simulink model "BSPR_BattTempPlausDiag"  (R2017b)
settings: Solver=FixedStepDiscrete  StartTime=0.0  StopTime=10.0  FixedStep=0.02  RelTol=1e-3  EnableMultiTasking=on
undefined symbols (not defined in the file): bin2dec, BSPR_cntBattTCnstErrDet_C, BSPR_cntBattTCnstErrHeal_C, BSPR_cntBattTHopErrDet_C, BSPR_cntBattTHopErrHeal_C, BSPR_cntBattTPlausDiag_CW, BSPR_cntCellTPlausDiag_CW, BSPR_cofBattTLowPassK_C, BSPR_tBattTCnstFaultThres_C, BSPR_tBattTempCnstHi_C, BSPR_tBattTempCnstLo_C, BSPR_tBattTempCnstThres_C, BSPR_tBattTempEnvtDiff_C, BSPR_tBattTHopFaultThres_C, BSPR_tBusbarTCnstFaultThres_C, BSPR_tBusbarTCnstHealThres_C, BSPR_tCellTCnstFaultThres_C, BSPR_tCellTCnstHealThres_C, BSPR_tiBattTCnstErrDet_C, BSPR_tiBattTCnstErrHeal_C
libraries: simulink x12
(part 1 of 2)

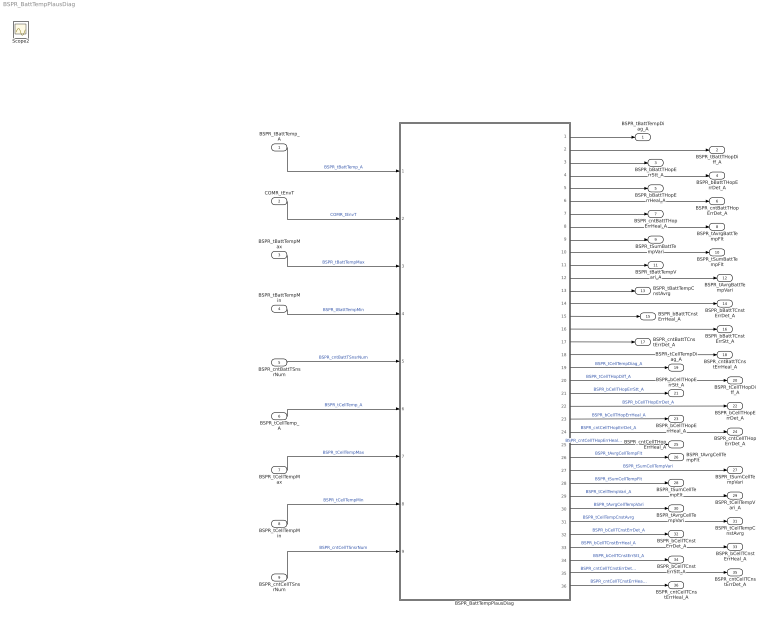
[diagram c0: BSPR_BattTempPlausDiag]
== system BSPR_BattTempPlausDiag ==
  BSPR_tBattTemp_A : Inport
  COMR_tEnvT : Inport  Port=2
  BSPR_tBattTempMax : Inport  Port=3
  BSPR_tBattTempMin : Inport  Port=4
  BSPR_cntBattTSnsrNum : Inport  Port=5
  BSPR_tCellTemp_A : Inport  Port=6
  BSPR_tCellTempMax : Inport  Port=7
  BSPR_tCellTempMin : Inport  Port=8
  BSPR_cntCellTSnsrNum : Inport  Port=9
  BSPR_BattTempPlausDiag : Subsystem
  BSPR_tBattTempDiag_A : Outport
  BSPR_tBattTHopDiff_A : Outport  Port=2
  BSPR_bBattTHopErrStt_A : Outport  Port=3
  BSPR_bBattTHopErrDet_A : Outport  Port=4
  BSPR_bBattTHopErrHeal_A : Outport  Port=5
  BSPR_cntBattTHopErrDet_A : Outport  Port=6
  BSPR_cntBattTHopErrHeal_A : Outport  Port=7
  BSPR_tAvrgBattTempFlt : Outport  Port=8
  BSPR_tSumBattTempVari : Outport  Port=9
  BSPR_tSumBattTempFlt : Outport  Port=10
  BSPR_tBattTempVari_A : Outport  Port=11
  BSPR_tAvrgBattTempVari : Outport  Port=12
  BSPR_tBattTempCnstAvrg : Outport  Port=13
  BSPR_bBattTCnstErrDet_A : Outport  Port=14
  BSPR_bBattTCnstErrHeal_A : Outport  Port=15
  BSPR_bBattTCnstErrStt_A : Outport  Port=16
  BSPR_cntBattTCnstErrDet_A : Outport  Port=17
  BSPR_cntBattTCnstErrHeal_A : Outport  Port=18
  BSPR_tCellTempDiag_A : Outport  Port=19  InitialOutput=[0]
  BSPR_tCellTHopDiff_A : Outport  Port=20  InitialOutput=[0]
  BSPR_bCellTHopErrStt_A : Outport  Port=21  InitialOutput=[0]
  BSPR_bCellTHopErrDet_A : Outport  Port=22
  BSPR_bCellTHopErrHeal_A : Outport  Port=23
  BSPR_cntCellTHopErrDet_A : Outport  Port=24  InitialOutput=[0]
  BSPR_cntCellTHopErrHeal_A : Outport  Port=25  InitialOutput=[0]
  BSPR_tAvrgCellTempFlt : Outport  Port=26  InitialOutput=[0]
  BSPR_tSumCellTempVari : Outport  Port=27  InitialOutput=[0]
  BSPR_tSumCellTempFlt : Outport  Port=28  InitialOutput=[0]
  BSPR_tCellTempVari_A : Outport  Port=29  InitialOutput=[0]
  BSPR_tAvrgCellTempVari : Outport  Port=30  InitialOutput=[0]
  BSPR_tCellTempCnstAvrg : Outport  Port=31  InitialOutput=[0]
  BSPR_bCellTCnstErrDet_A : Outport  Port=32  InitialOutput=[0]
  BSPR_bCellTCnstErrHeal_A : Outport  Port=33  InitialOutput=[0]
  BSPR_bCellTCnstErrStt_A : Outport  Port=34  InitialOutput=[0]
  BSPR_cntCellTCnstErrDet_A : Outport  Port=35  InitialOutput=[0]
  BSPR_cntCellTCnstErrHeal_A : Outport  Port=36  InitialOutput=[0]
  Scope2 : Scope
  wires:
  BSPR_tBattTemp_A/1 -> BSPR_BattTempPlausDiag/1(BSPR_tBattTemp_A)  "BSPR_tBattTemp_A"
  COMR_tEnvT/1 -> BSPR_BattTempPlausDiag/2(COMR_tEnvT)  "COMR_tEnvT"
  BSPR_tBattTempMax/1 -> BSPR_BattTempPlausDiag/3(BSPR_tBattTempMax)  "BSPR_tBattTempMax"
  BSPR_tBattTempMin/1 -> BSPR_BattTempPlausDiag/4(BSPR_tBattTempMin)  "BSPR_tBattTempMin"
  BSPR_BattTempPlausDiag/1(BSPR_tBattTempDiag_A) -> BSPR_tBattTempDiag_A/1
  BSPR_BattTempPlausDiag/2(BSPR_tBattTHopDiff_A) -> BSPR_tBattTHopDiff_A/1
  BSPR_BattTempPlausDiag/3(BSPR_bBattTHopErrStt_A) -> BSPR_bBattTHopErrStt_A/1
  BSPR_BattTempPlausDiag/4(BSPR_bBattTHopErrDet_A) -> BSPR_bBattTHopErrDet_A/1
  BSPR_BattTempPlausDiag/5(BSPR_bBattTHopErrHeal_A) -> BSPR_bBattTHopErrHeal_A/1
  BSPR_BattTempPlausDiag/6(BSPR_cntBattTHopErrDet_A) -> BSPR_cntBattTHopErrDet_A/1
  BSPR_BattTempPlausDiag/7(BSPR_cntBattTHopErrHeal_A) -> BSPR_cntBattTHopErrHeal_A/1
  BSPR_BattTempPlausDiag/8(BSPR_tAvrgBattTempFlt) -> BSPR_tAvrgBattTempFlt/1
  BSPR_BattTempPlausDiag/9(BSPR_tSumBattTempVari) -> BSPR_tSumBattTempVari/1
  BSPR_BattTempPlausDiag/10(BSPR_tSumBattTempFlt) -> BSPR_tSumBattTempFlt/1
  BSPR_BattTempPlausDiag/11(BSPR_tBattTempVari_A) -> BSPR_tBattTempVari_A/1
  BSPR_BattTempPlausDiag/12(BSPR_tAvrgBattTempVari) -> BSPR_tAvrgBattTempVari/1
  BSPR_BattTempPlausDiag/13(BSPR_tBattTempCnstAvrg) -> BSPR_tBattTempCnstAvrg/1
  BSPR_BattTempPlausDiag/14(BSPR_bBattTCnstErrDet_A) -> BSPR_bBattTCnstErrDet_A/1
  BSPR_BattTempPlausDiag/15(BSPR_bBattTCnstErrHeal_A) -> BSPR_bBattTCnstErrHeal_A/1
  BSPR_BattTempPlausDiag/16(BSPR_bBattTCnstErrStt_A) -> BSPR_bBattTCnstErrStt_A/1
  BSPR_BattTempPlausDiag/17(BSPR_cntBattTCnstErrDet_A) -> BSPR_cntBattTCnstErrDet_A/1
  BSPR_BattTempPlausDiag/18(BSPR_cntBattTCnstErrHeal_A) -> BSPR_cntBattTCnstErrHeal_A/1
  BSPR_cntBattTSnsrNum/1 -> BSPR_BattTempPlausDiag/5(BSPR_cntBattTSnsrNum)  "BSPR_cntBattTSnsrNum"
  BSPR_tCellTemp_A/1 -> BSPR_BattTempPlausDiag/6(BSPR_tCellTemp_A)  "BSPR_tCellTemp_A"
  BSPR_tCellTempMax/1 -> BSPR_BattTempPlausDiag/7(BSPR_tCellTempMax)  "BSPR_tCellTempMax"
  BSPR_tCellTempMin/1 -> BSPR_BattTempPlausDiag/8(BSPR_tCellTempMin)  "BSPR_tCellTempMin"
  BSPR_cntCellTSnsrNum/1 -> BSPR_BattTempPlausDiag/9(BSPR_cntCellTSnsrNum)  "BSPR_cntCellTSnsrNum"
  BSPR_BattTempPlausDiag/26(BSPR_tAvrgCellTempFlt) -> BSPR_tAvrgCellTempFlt/1  "BSPR_tAvrgCellTempFlt"
  BSPR_BattTempPlausDiag/30(BSPR_tAvrgCellTempVari) -> BSPR_tAvrgCellTempVari/1  "BSPR_tAvrgCellTempVari"
  BSPR_BattTempPlausDiag/23(BSPR_bCellTHopErrHeal_A) -> BSPR_bCellTHopErrHeal_A/1  "BSPR_bCellTHopErrHeal_A"
  BSPR_BattTempPlausDiag/32(BSPR_bCellTCnstErrDet_A) -> BSPR_bCellTCnstErrDet_A/1  "BSPR_bCellTCnstErrDet_A"
  BSPR_BattTempPlausDiag/36(BSPR_cntCellTCnstErrHeal_A) -> BSPR_cntCellTCnstErrHeal_A/1  "BSPR_cntCellTCnstErrHeal_A"
  BSPR_BattTempPlausDiag/33(BSPR_bCellTCnstErrHeal_A) -> BSPR_bCellTCnstErrHeal_A/1  "BSPR_bCellTCnstErrHeal_A"
  BSPR_BattTempPlausDiag/22(BSPR_bCellTHopErrDet_A) -> BSPR_bCellTHopErrDet_A/1  "BSPR_bCellTHopErrDet_A"
  BSPR_BattTempPlausDiag/29(BSPR_tCellTempVari_A) -> BSPR_tCellTempVari_A/1  "BSPR_tCellTempVari_A"
  BSPR_BattTempPlausDiag/34(BSPR_bCellTCnstErrStt_A) -> BSPR_bCellTCnstErrStt_A/1  "BSPR_bCellTCnstErrStt_A"
  BSPR_BattTempPlausDiag/31(BSPR_tCellTempCnstAvrg) -> BSPR_tCellTempCnstAvrg/1  "BSPR_tCellTempCnstAvrg"
  BSPR_BattTempPlausDiag/24(BSPR_cntCellTHopErrDet_A) -> BSPR_cntCellTHopErrDet_A/1  "BSPR_cntCellTHopErrDet_A"
  BSPR_BattTempPlausDiag/27(BSPR_tSumCellTempVari) -> BSPR_tSumCellTempVari/1  "BSPR_tSumCellTempVari"
  BSPR_BattTempPlausDiag/28(BSPR_tSumCellTempFlt) -> BSPR_tSumCellTempFlt/1  "BSPR_tSumCellTempFlt"
  BSPR_BattTempPlausDiag/35(BSPR_cntCellTCnstErrDet_A) -> BSPR_cntCellTCnstErrDet_A/1  "BSPR_cntCellTCnstErrDet_A"
  BSPR_BattTempPlausDiag/19(BSPR_tCellTempDiag_A) -> BSPR_tCellTempDiag_A/1  "BSPR_tCellTempDiag_A"
  BSPR_BattTempPlausDiag/25(BSPR_cntCellTHopErrHeal_A) -> BSPR_cntCellTHopErrHeal_A/1  "BSPR_cntCellTHopErrHeal_A"
  BSPR_BattTempPlausDiag/20(BSPR_tCellTHopDiff_A) -> BSPR_tCellTHopDiff_A/1  "BSPR_tCellTHopDiff_A"
  BSPR_BattTempPlausDiag/21(BSPR_bCellTHopErrStt_A) -> BSPR_bCellTHopErrStt_A/1  "BSPR_bCellTHopErrStt_A"

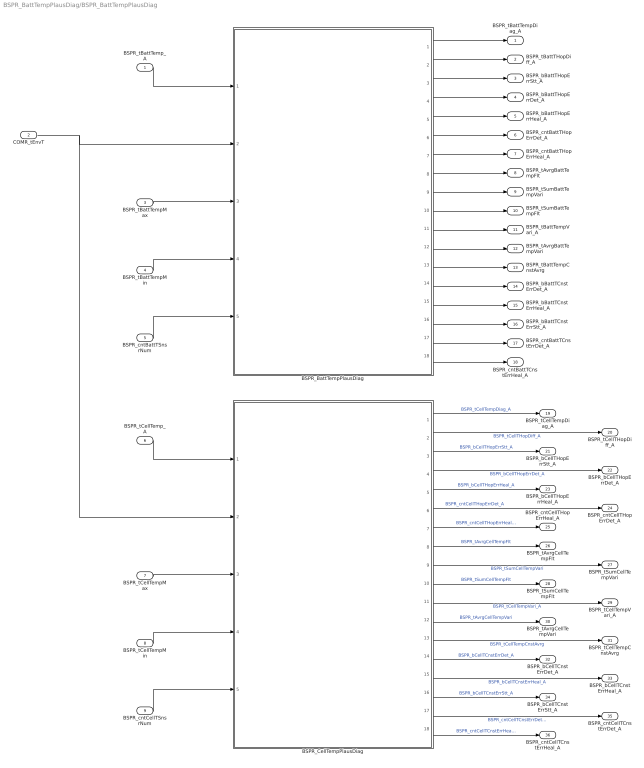
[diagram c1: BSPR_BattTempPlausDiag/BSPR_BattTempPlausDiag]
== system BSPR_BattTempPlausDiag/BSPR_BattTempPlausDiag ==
  BSPR_tBattTemp_A : Inport
  COMR_tEnvT : Inport  Port=2
  BSPR_tBattTempMax : Inport  Port=3
  BSPR_tBattTempMin : Inport  Port=4
  BSPR_cntBattTSnsrNum : Inport  Port=5
  BSPR_tCellTemp_A : Inport  Port=6
  BSPR_tCellTempMax : Inport  Port=7
  BSPR_tCellTempMin : Inport  Port=8
  BSPR_cntCellTSnsrNum : Inport  Port=9
  BSPR_BattTempPlausDiag : Subsystem
  BSPR_CellTempPlausDiag : Subsystem
  BSPR_tBattTempDiag_A : Outport
  BSPR_tBattTHopDiff_A : Outport  Port=2
  BSPR_bBattTHopErrStt_A : Outport  Port=3
  BSPR_bBattTHopErrDet_A : Outport  Port=4
  BSPR_bBattTHopErrHeal_A : Outport  Port=5
  BSPR_cntBattTHopErrDet_A : Outport  Port=6
  BSPR_cntBattTHopErrHeal_A : Outport  Port=7
  BSPR_tAvrgBattTempFlt : Outport  Port=8
  BSPR_tSumBattTempVari : Outport  Port=9
  BSPR_tSumBattTempFlt : Outport  Port=10
  BSPR_tBattTempVari_A : Outport  Port=11
  BSPR_tAvrgBattTempVari : Outport  Port=12
  BSPR_tBattTempCnstAvrg : Outport  Port=13
  BSPR_bBattTCnstErrDet_A : Outport  Port=14
  BSPR_bBattTCnstErrHeal_A : Outport  Port=15
  BSPR_bBattTCnstErrStt_A : Outport  Port=16
  BSPR_cntBattTCnstErrDet_A : Outport  Port=17
  BSPR_cntBattTCnstErrHeal_A : Outport  Port=18
  BSPR_tCellTempDiag_A : Outport  Port=19  InitialOutput=[0]
  BSPR_tCellTHopDiff_A : Outport  Port=20  InitialOutput=[0]
  BSPR_bCellTHopErrStt_A : Outport  Port=21  InitialOutput=[0]
  BSPR_bCellTHopErrDet_A : Outport  Port=22
  BSPR_bCellTHopErrHeal_A : Outport  Port=23
  BSPR_cntCellTHopErrDet_A : Outport  Port=24  InitialOutput=[0]
  BSPR_cntCellTHopErrHeal_A : Outport  Port=25  InitialOutput=[0]
  BSPR_tAvrgCellTempFlt : Outport  Port=26  InitialOutput=[0]
  BSPR_tSumCellTempVari : Outport  Port=27  InitialOutput=[0]
  BSPR_tSumCellTempFlt : Outport  Port=28  InitialOutput=[0]
  BSPR_tCellTempVari_A : Outport  Port=29  InitialOutput=[0]
  BSPR_tAvrgCellTempVari : Outport  Port=30  InitialOutput=[0]
  BSPR_tCellTempCnstAvrg : Outport  Port=31  InitialOutput=[0]
  BSPR_bCellTCnstErrDet_A : Outport  Port=32  InitialOutput=[0]
  BSPR_bCellTCnstErrHeal_A : Outport  Port=33  InitialOutput=[0]
  BSPR_bCellTCnstErrStt_A : Outport  Port=34  InitialOutput=[0]
  BSPR_cntCellTCnstErrDet_A : Outport  Port=35  InitialOutput=[0]
  BSPR_cntCellTCnstErrHeal_A : Outport  Port=36  InitialOutput=[0]
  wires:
  BSPR_tBattTemp_A/1 -> BSPR_BattTempPlausDiag/1(BSPR_tBattTemp_A)
  COMR_tEnvT/1 -> BSPR_CellTempPlausDiag/2(COMR_tEnvT), BSPR_BattTempPlausDiag/2(COMR_tEnvT)
  BSPR_tBattTempMax/1 -> BSPR_BattTempPlausDiag/3(BSPR_tBattTempMax)
  BSPR_tBattTempMin/1 -> BSPR_BattTempPlausDiag/4(BSPR_tBattTempMin)
  BSPR_cntBattTSnsrNum/1 -> BSPR_BattTempPlausDiag/5(BSPR_cntBattTSnsrNum)
  BSPR_BattTempPlausDiag/1(BSPR_tBattTempDiag_A) -> BSPR_tBattTempDiag_A/1
  BSPR_BattTempPlausDiag/2(BSPR_tBattTHopDiff_A) -> BSPR_tBattTHopDiff_A/1
  BSPR_BattTempPlausDiag/3(BSPR_bBattTHopErrStt_A) -> BSPR_bBattTHopErrStt_A/1
  BSPR_BattTempPlausDiag/4(BSPR_bBattTHopErrDet_A) -> BSPR_bBattTHopErrDet_A/1
  BSPR_BattTempPlausDiag/5(BSPR_bBattTHopErrHeal_A) -> BSPR_bBattTHopErrHeal_A/1
  BSPR_BattTempPlausDiag/6(BSPR_cntBattTHopErrDet_A) -> BSPR_cntBattTHopErrDet_A/1
  BSPR_BattTempPlausDiag/7(BSPR_cntBattTHopErrHeal_A) -> BSPR_cntBattTHopErrHeal_A/1
  BSPR_BattTempPlausDiag/8(BSPR_tAvrgBattTempFlt) -> BSPR_tAvrgBattTempFlt/1
  BSPR_BattTempPlausDiag/9(BSPR_tSumBattTempVari) -> BSPR_tSumBattTempVari/1
  BSPR_BattTempPlausDiag/10(BSPR_tSumBattTempFlt) -> BSPR_tSumBattTempFlt/1
  BSPR_BattTempPlausDiag/11(BSPR_tBattTempVari_A) -> BSPR_tBattTempVari_A/1
  BSPR_BattTempPlausDiag/12(BSPR_tAvrgBattTempVari) -> BSPR_tAvrgBattTempVari/1
  BSPR_BattTempPlausDiag/13(BSPR_tBattTempCnstAvrg) -> BSPR_tBattTempCnstAvrg/1
  BSPR_BattTempPlausDiag/14(BSPR_bBattTCnstErrDet_A) -> BSPR_bBattTCnstErrDet_A/1
  BSPR_BattTempPlausDiag/15(BSPR_bBattTCnstErrHeal_A) -> BSPR_bBattTCnstErrHeal_A/1
  BSPR_BattTempPlausDiag/16(BSPR_bBattTCnstErrStt_A) -> BSPR_bBattTCnstErrStt_A/1
  BSPR_BattTempPlausDiag/17(BSPR_cntBattTCnstErrDet_A) -> BSPR_cntBattTCnstErrDet_A/1
  BSPR_BattTempPlausDiag/18(BSPR_cntBattTCnstErrHeal_A) -> BSPR_cntBattTCnstErrHeal_A/1
  BSPR_cntCellTSnsrNum/1 -> BSPR_CellTempPlausDiag/5(BSPR_cntCellTSnsrNum)
  BSPR_tCellTempMin/1 -> BSPR_CellTempPlausDiag/4(BSPR_tCellTempMin)
  BSPR_tCellTempMax/1 -> BSPR_CellTempPlausDiag/3(BSPR_tCellTempMax)
  BSPR_tCellTemp_A/1 -> BSPR_CellTempPlausDiag/1(BSPR_tCellTemp_A)
  BSPR_CellTempPlausDiag/8(BSPR_tAvrgCellTempFlt) -> BSPR_tAvrgCellTempFlt/1  "BSPR_tAvrgCellTempFlt"
  BSPR_CellTempPlausDiag/15(BSPR_bCellTCnstErrHeal_A) -> BSPR_bCellTCnstErrHeal_A/1  "BSPR_bCellTCnstErrHeal_A"
  BSPR_CellTempPlausDiag/12(BSPR_tAvrgCellTempVari) -> BSPR_tAvrgCellTempVari/1  "BSPR_tAvrgCellTempVari"
  BSPR_CellTempPlausDiag/13(BSPR_tCellTempCnstAvrg) -> BSPR_tCellTempCnstAvrg/1  "BSPR_tCellTempCnstAvrg"
  BSPR_CellTempPlausDiag/11(BSPR_tCellTempVari_A) -> BSPR_tCellTempVari_A/1  "BSPR_tCellTempVari_A"
  BSPR_CellTempPlausDiag/16(BSPR_bCellTCnstErrStt_A) -> BSPR_bCellTCnstErrStt_A/1  "BSPR_bCellTCnstErrStt_A"
  BSPR_CellTempPlausDiag/4(BSPR_bCellTHopErrDet_A) -> BSPR_bCellTHopErrDet_A/1  "BSPR_bCellTHopErrDet_A"
  BSPR_CellTempPlausDiag/14(BSPR_bCellTCnstErrDet_A) -> BSPR_bCellTCnstErrDet_A/1  "BSPR_bCellTCnstErrDet_A"
  BSPR_CellTempPlausDiag/5(BSPR_bCellTHopErrHeal_A) -> BSPR_bCellTHopErrHeal_A/1  "BSPR_bCellTHopErrHeal_A"
  BSPR_CellTempPlausDiag/18(BSPR_cntCellTCnstErrHeal_A) -> BSPR_cntCellTCnstErrHeal_A/1  "BSPR_cntCellTCnstErrHeal_A"
  BSPR_CellTempPlausDiag/3(BSPR_bCellTHopErrStt_A) -> BSPR_bCellTHopErrStt_A/1  "BSPR_bCellTHopErrStt_A"
  BSPR_CellTempPlausDiag/7(BSPR_cntCellTHopErrHeal_A) -> BSPR_cntCellTHopErrHeal_A/1  "BSPR_cntCellTHopErrHeal_A"
  BSPR_CellTempPlausDiag/1(BSPR_tCellTempDiag_A) -> BSPR_tCellTempDiag_A/1  "BSPR_tCellTempDiag_A"
  BSPR_CellTempPlausDiag/6(BSPR_cntCellTHopErrDet_A) -> BSPR_cntCellTHopErrDet_A/1  "BSPR_cntCellTHopErrDet_A"
  BSPR_CellTempPlausDiag/9(BSPR_tSumCellTempVari) -> BSPR_tSumCellTempVari/1  "BSPR_tSumCellTempVari"
  BSPR_CellTempPlausDiag/2(BSPR_tCellTHopDiff_A) -> BSPR_tCellTHopDiff_A/1  "BSPR_tCellTHopDiff_A"
  BSPR_CellTempPlausDiag/10(BSPR_tSumCellTempFlt) -> BSPR_tSumCellTempFlt/1  "BSPR_tSumCellTempFlt"
  BSPR_CellTempPlausDiag/17(BSPR_cntCellTCnstErrDet_A) -> BSPR_cntCellTCnstErrDet_A/1  "BSPR_cntCellTCnstErrDet_A"

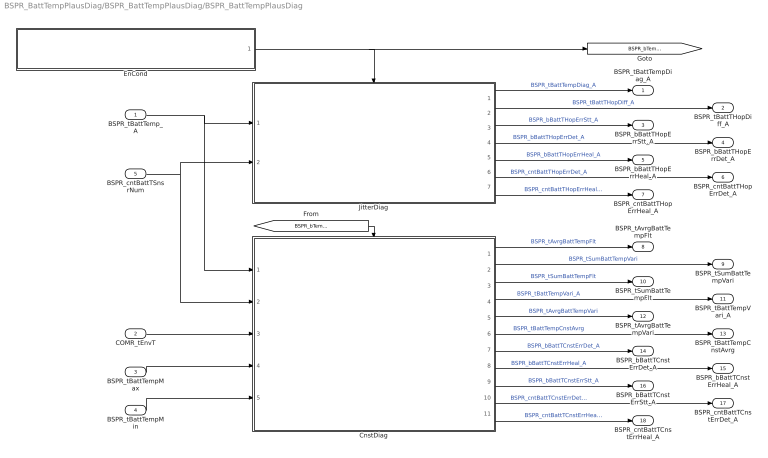
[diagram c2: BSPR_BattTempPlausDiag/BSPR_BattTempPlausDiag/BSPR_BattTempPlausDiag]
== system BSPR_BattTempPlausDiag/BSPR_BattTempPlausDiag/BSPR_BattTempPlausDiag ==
  BSPR_tBattTemp_A : Inport
  COMR_tEnvT : Inport  Port=2
  BSPR_tBattTempMax : Inport  Port=3
  BSPR_tBattTempMin : Inport  Port=4
  BSPR_cntBattTSnsrNum : Inport  Port=5
  CnstDiag : Subsystem
  EnCond : Subsystem
  JitterDiag : Subsystem
  BSPR_tBattTempDiag_A : Outport  InitialOutput=[0]
  BSPR_tBattTHopDiff_A : Outport  Port=2  InitialOutput=[0]
  BSPR_bBattTHopErrStt_A : Outport  Port=3  InitialOutput=[0]
  BSPR_bBattTHopErrDet_A : Outport  Port=4
  BSPR_bBattTHopErrHeal_A : Outport  Port=5
  BSPR_cntBattTHopErrDet_A : Outport  Port=6  InitialOutput=[0]
  BSPR_cntBattTHopErrHeal_A : Outport  Port=7  InitialOutput=[0]
  BSPR_tAvrgBattTempFlt : Outport  Port=8  InitialOutput=[0]
  BSPR_tSumBattTempVari : Outport  Port=9  InitialOutput=[0]
  BSPR_tSumBattTempFlt : Outport  Port=10  InitialOutput=[0]
  BSPR_tBattTempVari_A : Outport  Port=11  InitialOutput=[0]
  BSPR_tAvrgBattTempVari : Outport  Port=12  InitialOutput=[0]
  BSPR_tBattTempCnstAvrg : Outport  Port=13  InitialOutput=[0]
  BSPR_bBattTCnstErrDet_A : Outport  Port=14  InitialOutput=[0]
  BSPR_bBattTCnstErrHeal_A : Outport  Port=15  InitialOutput=[0]
  BSPR_bBattTCnstErrStt_A : Outport  Port=16  InitialOutput=[0]
  BSPR_cntBattTCnstErrDet_A : Outport  Port=17  InitialOutput=[0]
  BSPR_cntBattTCnstErrHeal_A : Outport  Port=18  InitialOutput=[0]
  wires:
  CnstDiag/4(BSPR_tBattTempVari_A) -> BSPR_tBattTempVari_A/1  "BSPR_tBattTempVari_A"
  JitterDiag/1(BSPR_tBattTempDiag_A) -> BSPR_tBattTempDiag_A/1  "BSPR_tBattTempDiag_A"
  CnstDiag/8(BSPR_bBattTCnstErrHeal_A) -> BSPR_bBattTCnstErrHeal_A/1  "BSPR_bBattTCnstErrHeal_A"
  CnstDiag/1(BSPR_tAvrgBattTempFlt) -> BSPR_tAvrgBattTempFlt/1  "BSPR_tAvrgBattTempFlt"
  CnstDiag/11(BSPR_cntBattTCnstErrHeal_A) -> BSPR_cntBattTCnstErrHeal_A/1  "BSPR_cntBattTCnstErrHeal_A"
  JitterDiag/7(BSPR_cntBattTHopErrHeal_A) -> BSPR_cntBattTHopErrHeal_A/1  "BSPR_cntBattTHopErrHeal_A"
  CnstDiag/9(BSPR_bBattTCnstErrStt_A) -> BSPR_bBattTCnstErrStt_A/1  "BSPR_bBattTCnstErrStt_A"
  CnstDiag/10(BSPR_cntBattTCnstErrDet_A) -> BSPR_cntBattTCnstErrDet_A/1  "BSPR_cntBattTCnstErrDet_A"
  COMR_tEnvT/1 -> CnstDiag/3(COMR_tEnvT)
  BSPR_tBattTemp_A/1 -> CnstDiag/1(BSPR_tBattTemp_A), JitterDiag/1(BSPR_tBattTemp_A)
  JitterDiag/6(BSPR_cntBattTHopErrDet_A) -> BSPR_cntBattTHopErrDet_A/1  "BSPR_cntBattTHopErrDet_A"
  BSPR_tBattTempMin/1 -> CnstDiag/5(BSPR_tBattTempMin)
  JitterDiag/3(BSPR_bBattTHopErrStt_A) -> BSPR_bBattTHopErrStt_A/1  "BSPR_bBattTHopErrStt_A"
  JitterDiag/4(BSPR_bBattTHopErrDet_A) -> BSPR_bBattTHopErrDet_A/1  "BSPR_bBattTHopErrDet_A"
  JitterDiag/5(BSPR_bBattTHopErrHeal_A) -> BSPR_bBattTHopErrHeal_A/1  "BSPR_bBattTHopErrHeal_A"
  JitterDiag/2(BSPR_tBattTHopDiff_A) -> BSPR_tBattTHopDiff_A/1  "BSPR_tBattTHopDiff_A"
  BSPR_cntBattTSnsrNum/1 -> JitterDiag/2(BSPR_cntBattTSnsrNum), CnstDiag/2(BSPR_cntBattTSnsrNum)
  CnstDiag/6(BSPR_tBattTempCnstAvrg) -> BSPR_tBattTempCnstAvrg/1  "BSPR_tBattTempCnstAvrg"
  CnstDiag/7(BSPR_bBattTCnstErrDet_A) -> BSPR_bBattTCnstErrDet_A/1  "BSPR_bBattTCnstErrDet_A"
  CnstDiag/2(BSPR_tSumBattTempVari) -> BSPR_tSumBattTempVari/1  "BSPR_tSumBattTempVari"
  CnstDiag/3(BSPR_tSumBattTempFlt) -> BSPR_tSumBattTempFlt/1  "BSPR_tSumBattTempFlt"
  CnstDiag/5(BSPR_tAvrgBattTempVari) -> BSPR_tAvrgBattTempVari/1  "BSPR_tAvrgBattTempVari"
  BSPR_tBattTempMax/1 -> CnstDiag/4(BSPR_tBattTempMax)
  EnCond/1(BSPR_bTempPlausDiagEn) -> JitterDiag/Enable, [BSPR_bTempPlausDiagEn]
  [BSPR_bTempPlausDiagEn] -> CnstDiag/Enable

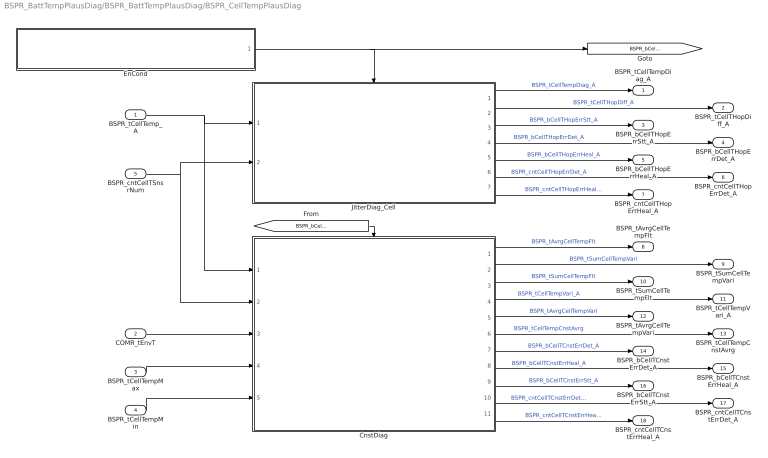
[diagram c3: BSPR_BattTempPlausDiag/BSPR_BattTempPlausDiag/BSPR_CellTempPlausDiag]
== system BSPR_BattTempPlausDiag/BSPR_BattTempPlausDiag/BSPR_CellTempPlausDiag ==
  BSPR_tCellTemp_A : Inport
  COMR_tEnvT : Inport  Port=2
  BSPR_tCellTempMax : Inport  Port=3
  BSPR_tCellTempMin : Inport  Port=4
  BSPR_cntCellTSnsrNum : Inport  Port=5
  CnstDiag : Subsystem
  EnCond : Subsystem
  JitterDiag_Cell : Subsystem
  BSPR_tCellTempDiag_A : Outport  InitialOutput=[0]
  BSPR_tCellTHopDiff_A : Outport  Port=2  InitialOutput=[0]
  BSPR_bCellTHopErrStt_A : Outport  Port=3  InitialOutput=[0]
  BSPR_bCellTHopErrDet_A : Outport  Port=4
  BSPR_bCellTHopErrHeal_A : Outport  Port=5
  BSPR_cntCellTHopErrDet_A : Outport  Port=6  InitialOutput=[0]
  BSPR_cntCellTHopErrHeal_A : Outport  Port=7  InitialOutput=[0]
  BSPR_tAvrgCellTempFlt : Outport  Port=8  InitialOutput=[0]
  BSPR_tSumCellTempVari : Outport  Port=9  InitialOutput=[0]
  BSPR_tSumCellTempFlt : Outport  Port=10  InitialOutput=[0]
  BSPR_tCellTempVari_A : Outport  Port=11  InitialOutput=[0]
  BSPR_tAvrgCellTempVari : Outport  Port=12  InitialOutput=[0]
  BSPR_tCellTempCnstAvrg : Outport  Port=13  InitialOutput=[0]
  BSPR_bCellTCnstErrDet_A : Outport  Port=14  InitialOutput=[0]
  BSPR_bCellTCnstErrHeal_A : Outport  Port=15  InitialOutput=[0]
  BSPR_bCellTCnstErrStt_A : Outport  Port=16  InitialOutput=[0]
  BSPR_cntCellTCnstErrDet_A : Outport  Port=17  InitialOutput=[0]
  BSPR_cntCellTCnstErrHeal_A : Outport  Port=18  InitialOutput=[0]
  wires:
  [BSPR_bCellTempPlausDiagEn] -> CnstDiag/Enable
  EnCond/1(BSPR_bCellTempPlausDiagEn) -> [BSPR_bCellTempPlausDiagEn], JitterDiag_Cell/Enable
  BSPR_tCellTempMax/1 -> CnstDiag/4(BSPR_tCellTempMax)
  CnstDiag/5(BSPR_tAvrgCellTempVari) -> BSPR_tAvrgCellTempVari/1  "BSPR_tAvrgCellTempVari"
  CnstDiag/3(BSPR_tSumCellTempFlt) -> BSPR_tSumCellTempFlt/1  "BSPR_tSumCellTempFlt"
  CnstDiag/2(BSPR_tSumCellTempVari) -> BSPR_tSumCellTempVari/1  "BSPR_tSumCellTempVari"
  CnstDiag/7(BSPR_bCellTCnstErrDet_A) -> BSPR_bCellTCnstErrDet_A/1  "BSPR_bCellTCnstErrDet_A"
  CnstDiag/6(BSPR_tCellTempCnstAvrg) -> BSPR_tCellTempCnstAvrg/1  "BSPR_tCellTempCnstAvrg"
  BSPR_cntCellTSnsrNum/1 -> CnstDiag/2(BSPR_cntCellTSnsrNum), JitterDiag_Cell/2(BSPR_cntCellTSnsrNum)
  JitterDiag_Cell/2(BSPR_tCellTHopDiff_A) -> BSPR_tCellTHopDiff_A/1  "BSPR_tCellTHopDiff_A"
  JitterDiag_Cell/5(BSPR_bCellTHopErrHeal_A) -> BSPR_bCellTHopErrHeal_A/1  "BSPR_bCellTHopErrHeal_A"
  JitterDiag_Cell/4(BSPR_bCellTHopErrDet_A) -> BSPR_bCellTHopErrDet_A/1  "BSPR_bCellTHopErrDet_A"
  JitterDiag_Cell/3(BSPR_bCellTHopErrStt_A) -> BSPR_bCellTHopErrStt_A/1  "BSPR_bCellTHopErrStt_A"
  BSPR_tCellTempMin/1 -> CnstDiag/5(BSPR_tCellTempMin)
  JitterDiag_Cell/6(BSPR_cntCellTHopErrDet_A) -> BSPR_cntCellTHopErrDet_A/1  "BSPR_cntCellTHopErrDet_A"
  BSPR_tCellTemp_A/1 -> JitterDiag_Cell/1(BSPR_tCellTemp_A), CnstDiag/1(BSPR_tCellTemp_A)
  COMR_tEnvT/1 -> CnstDiag/3(COMR_tEnvT)
  CnstDiag/10(BSPR_cntCellTCnstErrDet_A) -> BSPR_cntCellTCnstErrDet_A/1  "BSPR_cntCellTCnstErrDet_A"
  CnstDiag/9(BSPR_bCellTCnstErrStt_A) -> BSPR_bCellTCnstErrStt_A/1  "BSPR_bCellTCnstErrStt_A"
  JitterDiag_Cell/7(BSPR_cntBattTHopErrHeal_A) -> BSPR_cntCellTHopErrHeal_A/1  "BSPR_cntCellTHopErrHeal_A"
  CnstDiag/11(BSPR_cntCellTCnstErrHeal_A) -> BSPR_cntCellTCnstErrHeal_A/1  "BSPR_cntCellTCnstErrHeal_A"
  CnstDiag/1(BSPR_tAvrgCellTempFlt) -> BSPR_tAvrgCellTempFlt/1  "BSPR_tAvrgCellTempFlt"
  CnstDiag/8(BSPR_bCellTCnstErrHeal_A) -> BSPR_bCellTCnstErrHeal_A/1  "BSPR_bCellTCnstErrHeal_A"
  JitterDiag_Cell/1(BSPR_tCellTempDiag_A) -> BSPR_tCellTempDiag_A/1  "BSPR_tCellTempDiag_A"
  CnstDiag/4(BSPR_tCellTempVari_A) -> BSPR_tCellTempVari_A/1  "BSPR_tCellTempVari_A"

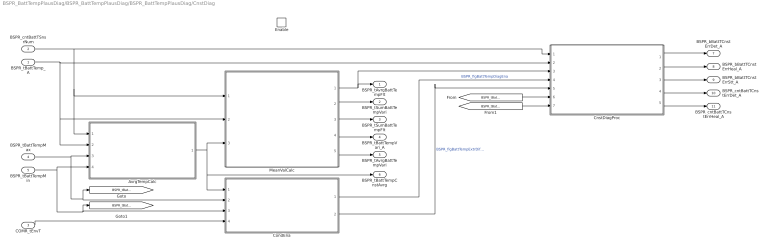
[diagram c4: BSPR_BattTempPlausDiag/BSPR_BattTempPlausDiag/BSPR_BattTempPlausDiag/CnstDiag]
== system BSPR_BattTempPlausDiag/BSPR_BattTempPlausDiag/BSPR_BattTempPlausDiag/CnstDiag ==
  BSPR_tBattTemp_A : Inport
  BSPR_cntBattTSnsrNum : Inport  Port=2
  COMR_tEnvT : Inport  Port=3
  BSPR_tBattTempMax : Inport  Port=4
  BSPR_tBattTempMin : Inport  Port=5
  Enable : EnablePort  StatesWhenEnabling=reset
  AvrgTempCalc : Subsystem
  CnstDiagProc : Subsystem
  CondEna : Subsystem
  MeanValCalc : Subsystem
  BSPR_tAvrgBattTempFlt : Outport  InitialOutput=[0]
  BSPR_tSumBattTempVari : Outport  Port=2  InitialOutput=[0]
  BSPR_tSumBattTempFlt : Outport  Port=3  InitialOutput=[0]
  BSPR_tBattTempVari_A : Outport  Port=4  InitialOutput=[0]
  BSPR_tAvrgBattTempVari : Outport  Port=5  InitialOutput=[0]
  BSPR_tBattTempCnstAvrg : Outport  Port=6
  BSPR_bBattTCnstErrDet_A : Outport  Port=7  InitialOutput=[0]
  BSPR_bBattTCnstErrHeal_A : Outport  Port=8  InitialOutput=[0]
  BSPR_bBattTCnstErrStt_A : Outport  Port=9  InitialOutput=[0]
  BSPR_cntBattTCnstErrDet_A : Outport  Port=10  InitialOutput=[0]
  BSPR_cntBattTCnstErrHeal_A : Outport  Port=11  InitialOutput=[0]
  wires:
  MeanValCalc/5(BSPR_tAvrgBattTempVari) -> BSPR_tAvrgBattTempVari/1
  AvrgTempCalc/1(BSPR_tBattTempCnstAvrg) -> MeanValCalc/3(BSPR_tBattTempCnstAvrg), BSPR_tBattTempCnstAvrg/1, CondEna/1(BSPR_tBattTempCnstAvrg)
  MeanValCalc/3(BSPR_tSumBattTempFlt) -> BSPR_tSumBattTempFlt/1
  MeanValCalc/2(BSPR_tSumBattTempVari) -> BSPR_tSumBattTempVari/1
  MeanValCalc/4(BSPR_tBattTempVari_A) -> BSPR_tBattTempVari_A/1
  CnstDiagProc/5(BSPR_cntBattTCnstErrHeal_A) -> BSPR_cntBattTCnstErrHeal_A/1
  CnstDiagProc/1(BSPR_bBattTCnstErrDet_A) -> BSPR_bBattTCnstErrDet_A/1
  BSPR_tBattTempMax/1 -> AvrgTempCalc/3(BSPR_tBattTempMax), [BSPR_tBattTempMax], CondEna/2(BSPR_tBattTempMax)
  BSPR_tBattTempMin/1 -> [BSPR_tBattTempMin], CondEna/3(BSPR_tBattTempMin), AvrgTempCalc/4(BSPR_tBattTempMin)
  COMR_tEnvT/1 -> CondEna/4(COMR_tEnvT)
  BSPR_tBattTemp_A/1 -> CnstDiagProc/2(BSPR_tBattTemp_A), MeanValCalc/2(BSPR_tBattTemp_A), AvrgTempCalc/2(BSPR_tBattTemp_A)
  CnstDiagProc/2(BSPR_bBattTCnstErrHeal_A) -> BSPR_bBattTCnstErrHeal_A/1
  CnstDiagProc/3(BSPR_bBattTCnstErrStt_A) -> BSPR_bBattTCnstErrStt_A/1
  CnstDiagProc/4(BSPR_cntBattTCnstErrDet_A) -> BSPR_cntBattTCnstErrDet_A/1
  MeanValCalc/1(BSPR_tAvrgBattTempFlt) -> CnstDiagProc/3(BSPR_tAvrgBattTempFlt), BSPR_tAvrgBattTempFlt/1
  CondEna/1(BSPR_flgBattTempDiagEna) -> CnstDiagProc/4(BSPR_flgBattTempDiagEna)  "BSPR_flgBattTempDiagEna"
  CondEna/2(BSPR_flgBattTempExtrDiffEna) -> CnstDiagProc/5(BSPR_flgBattTempExtrDiffEna)  "BSPR_flgBattTempExtrDiffEna"
  BSPR_cntBattTSnsrNum/1 -> CnstDiagProc/1(BSPR_cntBattTSnsrNum), MeanValCalc/1(BSPR_cntBattTSnsrNum), AvrgTempCalc/1(BSPR_cntBattTSnsrNum)
  [BSPR_tBattTempMax] -> CnstDiagProc/6(BSPR_tBattTempMax)
  [BSPR_tBattTempMin] -> CnstDiagProc/7(BSPR_tBattTempMin)

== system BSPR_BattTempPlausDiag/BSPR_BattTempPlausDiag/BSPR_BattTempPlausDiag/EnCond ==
  Constant : Constant  Value=5  OutDataTypeStr=single
  Constant1 : Constant  OutDataTypeStr=boolean
  TONV_100msTimeDebounce : Subsystem  TreatAsAtomicUnit=on  RTWFcnName=TONV_100msTimeDebounce  RTWFileName=SrvLib
  BSPR_bTempPlausDiagEn : Outport
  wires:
  TONV_100msTimeDebounce/1(y) -> BSPR_bTempPlausDiagEn/1  "BSPR_bTempPlausDiagEn"
  Constant/1 -> TONV_100msTimeDebounce/2(T)
  Constant1/1 -> TONV_100msTimeDebounce/1(u)

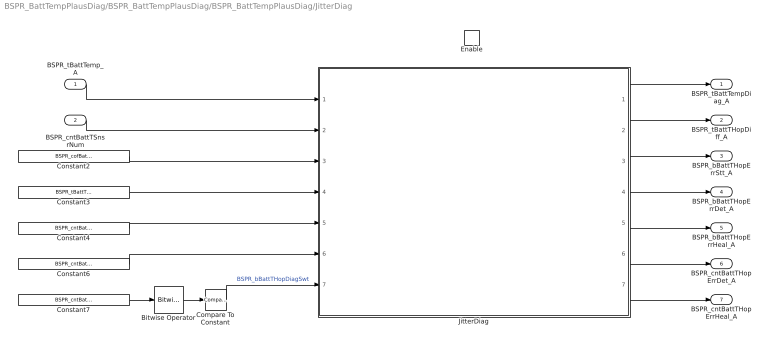
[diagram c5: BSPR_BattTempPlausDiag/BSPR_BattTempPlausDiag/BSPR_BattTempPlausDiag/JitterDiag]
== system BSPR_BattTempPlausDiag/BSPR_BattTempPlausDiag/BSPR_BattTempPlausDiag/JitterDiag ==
  BSPR_tBattTemp_A : Inport
  BSPR_cntBattTSnsrNum : Inport  Port=2
  Enable : EnablePort  StatesWhenEnabling=reset
  Bitwise Operator : simulink/Logic and Bit Operations/Bitwise Operator  logicop=AND  UseBitMask=on  BitMask=bin2dec('00000001')  BitMaskRealWorld=Stored Integer
  Compare To Constant : simulink/Logic and Bit Operations/Compare To Constant  relop===  const=1  OutDataTypeStr=boolean
  Constant2 : Constant  Value=BSPR_cofBattTLowPassK_C
  Constant3 : Constant  Value=BSPR_tBattTHopFaultThres_C
  Constant4 : Constant  Value=BSPR_cntBattTHopErrDet_C
  Constant6 : Constant  Value=BSPR_cntBattTHopErrHeal_C
  Constant7 : Constant  Value=BSPR_cntBattTPlausDiag_CW
  JitterDiag : Stateflow chart  TreatAsAtomicUnit=on
  BSPR_tBattTempDiag_A : Outport  InitialOutput=[0]
  BSPR_tBattTHopDiff_A : Outport  Port=2  InitialOutput=[0]
  BSPR_bBattTHopErrStt_A : Outport  Port=3  InitialOutput=[0]
  BSPR_bBattTHopErrDet_A : Outport  Port=4  InitialOutput=[0]
  BSPR_bBattTHopErrHeal_A : Outport  Port=5  InitialOutput=[0]
  BSPR_cntBattTHopErrDet_A : Outport  Port=6  InitialOutput=[0]
  BSPR_cntBattTHopErrHeal_A : Outport  Port=7  InitialOutput=[0]
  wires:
  BSPR_cntBattTSnsrNum/1 -> JitterDiag/2(BSPR_cntBattTSnsrNum)
  Constant2/1 -> JitterDiag/3(BSPR_cofBattTLowPassK_C)
  Constant3/1 -> JitterDiag/4(BSPR_tBattTHopFaultThres_C)
  Constant4/1 -> JitterDiag/5(BSPR_cntBattTHopErrDet_C)
  Constant6/1 -> JitterDiag/6(BSPR_cntBattTHopErrHeal_C)
  BSPR_tBattTemp_A/1 -> JitterDiag/1(BSPR_tBattTemp_A)
  JitterDiag/3(BSPR_bBattTHopErrStt_A) -> BSPR_bBattTHopErrStt_A/1
  JitterDiag/2(BSPR_tBattTHopDiff_A) -> BSPR_tBattTHopDiff_A/1
  JitterDiag/1(BSPR_tBattTempDiag_A) -> BSPR_tBattTempDiag_A/1
  JitterDiag/4(BSPR_bBattTHopErrDet_A) -> BSPR_bBattTHopErrDet_A/1
  JitterDiag/5(BSPR_bBattTHopErrHeal_A) -> BSPR_bBattTHopErrHeal_A/1
  JitterDiag/6(BSPR_cntBattTHopErrDet_A) -> BSPR_cntBattTHopErrDet_A/1
  JitterDiag/7(BSPR_cntBattTHopErrHeal_A) -> BSPR_cntBattTHopErrHeal_A/1
  Compare To Constant/1 -> JitterDiag/7(BSPR_bBattTHopDiagSwt)  "BSPR_bBattTHopDiagSwt"
  Bitwise Operator/1 -> Compare To Constant/1
  Constant7/1 -> Bitwise Operator/1

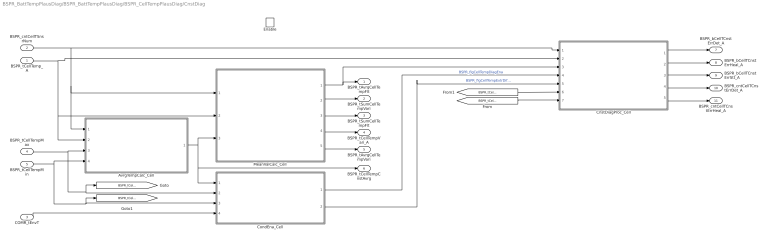
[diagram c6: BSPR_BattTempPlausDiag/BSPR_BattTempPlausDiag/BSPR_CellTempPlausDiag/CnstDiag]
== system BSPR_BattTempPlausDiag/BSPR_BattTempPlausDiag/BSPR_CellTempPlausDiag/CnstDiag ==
  BSPR_tCellTemp_A : Inport
  BSPR_cntCellTSnsrNum : Inport  Port=2
  COMR_tEnvT : Inport  Port=3
  BSPR_tCellTempMax : Inport  Port=4
  BSPR_tCellTempMin : Inport  Port=5
  Enable : EnablePort  StatesWhenEnabling=reset
  AvrgTempCalc_Cell : Subsystem
  CnstDiagProc_Cell : Subsystem
  CondEna_Cell : Subsystem
  MeanValCalc_Cell : Subsystem
  BSPR_tAvrgCellTempFlt : Outport  InitialOutput=[0]
  BSPR_tSumCellTempVari : Outport  Port=2  InitialOutput=[0]
  BSPR_tSumCellTempFlt : Outport  Port=3  InitialOutput=[0]
  BSPR_tCellTempVari_A : Outport  Port=4  InitialOutput=[0]
  BSPR_tAvrgCellTempVari : Outport  Port=5  InitialOutput=[0]
  BSPR_tCellTempCnstAvrg : Outport  Port=6
  BSPR_bCellTCnstErrDet_A : Outport  Port=7  InitialOutput=[0]
  BSPR_bCellTCnstErrHeal_A : Outport  Port=8  InitialOutput=[0]
  BSPR_bCellTCnstErrStt_A : Outport  Port=9  InitialOutput=[0]
  BSPR_cntCellTCnstErrDet_A : Outport  Port=10  InitialOutput=[0]
  BSPR_cntCellTCnstErrHeal_A : Outport  Port=11  InitialOutput=[0]
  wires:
  BSPR_cntCellTSnsrNum/1 -> AvrgTempCalc_Cell/1(BSPR_cntCellTSnsrNum), MeanValCalc_Cell/1(BSPR_cntCellTSnsrNum), CnstDiagProc_Cell/1(BSPR_cntCellTSnsrNum)
  CondEna_Cell/2(BSPR_flgCellTempExtrDiffEna) -> CnstDiagProc_Cell/5(BSPR_flgCellTempExtrDiffEna)  "BSPR_flgCellTempExtrDiffEna"
  CondEna_Cell/1(BSPR_flgCellTempDiagEna) -> CnstDiagProc_Cell/4(BSPR_flgCellTempDiagEna)  "BSPR_flgCellTempDiagEna"
  MeanValCalc_Cell/1(BSPR_tAvrgCellTempFlt) -> BSPR_tAvrgCellTempFlt/1, CnstDiagProc_Cell/3(BSPR_tAvrgCellTempFlt)
  CnstDiagProc_Cell/4(BSPR_cntCellTCnstErrDet_A) -> BSPR_cntCellTCnstErrDet_A/1
  CnstDiagProc_Cell/3(BSPR_bCellTCnstErrStt_A) -> BSPR_bCellTCnstErrStt_A/1
  CnstDiagProc_Cell/2(BSPR_bCellTCnstErrHeal_A) -> BSPR_bCellTCnstErrHeal_A/1
  BSPR_tCellTemp_A/1 -> AvrgTempCalc_Cell/2(BSPR_tCellTemp_A), MeanValCalc_Cell/2(BSPR_tCellTemp_A), CnstDiagProc_Cell/2(BSPR_tCellTemp_A)
  COMR_tEnvT/1 -> CondEna_Cell/4(COMR_tEnvT)
  BSPR_tCellTempMin/1 -> AvrgTempCalc_Cell/4(BSPR_tCellTempMin), [BSPR_tCellTempMin], CondEna_Cell/3(BSPR_tCellTempMin)
  BSPR_tCellTempMax/1 -> [BSPR_tCellTempMax], CondEna_Cell/2(BSPR_tCellTempMax), AvrgTempCalc_Cell/3(BSPR_tCellTempMax)
  CnstDiagProc_Cell/1(BSPR_bCellTCnstErrDet_A) -> BSPR_bCellTCnstErrDet_A/1
  CnstDiagProc_Cell/5(BSPR_cntCellTCnstErrHeal_A) -> BSPR_cntCellTCnstErrHeal_A/1
  MeanValCalc_Cell/4(BSPR_tCellTempVari_A) -> BSPR_tCellTempVari_A/1
  MeanValCalc_Cell/2(BSPR_tSumCellTempVari) -> BSPR_tSumCellTempVari/1
  MeanValCalc_Cell/3(BSPR_tSumCellTempFlt) -> BSPR_tSumCellTempFlt/1
  AvrgTempCalc_Cell/1(BSPR_tCellTempCnstAvrg) -> CondEna_Cell/1(BSPR_tCellTempCnstAvrg), BSPR_tCellTempCnstAvrg/1, MeanValCalc_Cell/3(BSPR_tCellTempCnstAvrg)
  MeanValCalc_Cell/5(BSPR_tAvrgCellTempVari) -> BSPR_tAvrgCellTempVari/1
  [BSPR_tCellTempMin] -> CnstDiagProc_Cell/7(BSPR_tCellTempMin)
  [BSPR_tCellTempMax] -> CnstDiagProc_Cell/6(BSPR_tCellTempMax)

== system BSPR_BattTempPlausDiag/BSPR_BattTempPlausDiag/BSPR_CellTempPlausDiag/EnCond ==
  Constant : Constant  Value=5  OutDataTypeStr=single
  Constant1 : Constant  OutDataTypeStr=boolean
  TONV_100msTimeDebounce : Subsystem  TreatAsAtomicUnit=on  RTWFcnName=TONV_100msTimeDebounce  RTWFileName=SrvLib
  BSPR_bCellTempPlausDiagEn : Outport
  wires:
  Constant1/1 -> TONV_100msTimeDebounce/1(u)
  Constant/1 -> TONV_100msTimeDebounce/2(T)
  TONV_100msTimeDebounce/1(y) -> BSPR_bCellTempPlausDiagEn/1  "BSPR_bCellTempPlausDiagEn"

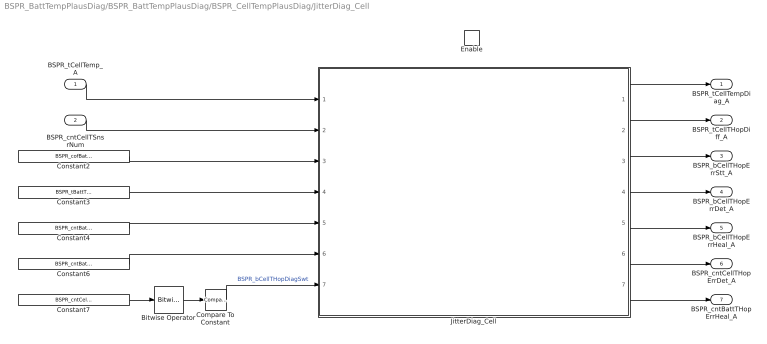
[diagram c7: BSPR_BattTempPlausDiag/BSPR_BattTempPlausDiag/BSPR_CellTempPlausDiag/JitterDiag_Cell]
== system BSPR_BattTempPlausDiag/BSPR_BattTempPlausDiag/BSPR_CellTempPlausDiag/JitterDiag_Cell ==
  BSPR_tCellTemp_A : Inport
  BSPR_cntCellTSnsrNum : Inport  Port=2
  Enable : EnablePort  StatesWhenEnabling=reset
  Bitwise Operator : simulink/Logic and Bit Operations/Bitwise Operator  logicop=AND  UseBitMask=on  BitMask=bin2dec('00000001')  BitMaskRealWorld=Stored Integer
  Compare To Constant : simulink/Logic and Bit Operations/Compare To Constant  relop===  const=1  OutDataTypeStr=boolean
  Constant2 : Constant  Value=BSPR_cofBattTLowPassK_C
  Constant3 : Constant  Value=BSPR_tBattTHopFaultThres_C
  Constant4 : Constant  Value=BSPR_cntBattTHopErrDet_C
  Constant6 : Constant  Value=BSPR_cntBattTHopErrHeal_C
  Constant7 : Constant  Value=BSPR_cntCellTPlausDiag_CW
  JitterDiag_Cell : Stateflow chart  TreatAsAtomicUnit=on
  BSPR_tCellTempDiag_A : Outport  InitialOutput=[0]
  BSPR_tCellTHopDiff_A : Outport  Port=2  InitialOutput=[0]
  BSPR_bCellTHopErrStt_A : Outport  Port=3  InitialOutput=[0]
  BSPR_bCellTHopErrDet_A : Outport  Port=4  InitialOutput=[0]
  BSPR_bCellTHopErrHeal_A : Outport  Port=5  InitialOutput=[0]
  BSPR_cntCellTHopErrDet_A : Outport  Port=6  InitialOutput=[0]
  BSPR_cntBattTHopErrHeal_A : Outport  Port=7  InitialOutput=[0]
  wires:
  Constant7/1 -> Bitwise Operator/1
  Bitwise Operator/1 -> Compare To Constant/1
  Compare To Constant/1 -> JitterDiag_Cell/7(BSPR_bBattTHopDiagSwt)  "BSPR_bCellTHopDiagSwt"
  JitterDiag_Cell/7(BSPR_cntBattTHopErrHeal_A) -> BSPR_cntBattTHopErrHeal_A/1
  JitterDiag_Cell/6(BSPR_cntBattTHopErrDet_A) -> BSPR_cntCellTHopErrDet_A/1
  JitterDiag_Cell/5(BSPR_bBattTHopErrHeal_A) -> BSPR_bCellTHopErrHeal_A/1
  JitterDiag_Cell/4(BSPR_bBattTHopErrDet_A) -> BSPR_bCellTHopErrDet_A/1
  JitterDiag_Cell/1(BSPR_tBattTempDiag_A) -> BSPR_tCellTempDiag_A/1
  JitterDiag_Cell/2(BSPR_tBattTHopDiff_A) -> BSPR_tCellTHopDiff_A/1
  JitterDiag_Cell/3(BSPR_bBattTHopErrStt_A) -> BSPR_bCellTHopErrStt_A/1
  BSPR_tCellTemp_A/1 -> JitterDiag_Cell/1(BSPR_tBattTemp_A)
  Constant6/1 -> JitterDiag_Cell/6(BSPR_cntBattTHopErrHeal_C)
  Constant4/1 -> JitterDiag_Cell/5(BSPR_cntBattTHopErrDet_C)
  Constant3/1 -> JitterDiag_Cell/4(BSPR_tBattTHopFaultThres_C)
  Constant2/1 -> JitterDiag_Cell/3(BSPR_cofBattTLowPassK_C)
  BSPR_cntCellTSnsrNum/1 -> JitterDiag_Cell/2(BSPR_cntBattTSnsrNum)

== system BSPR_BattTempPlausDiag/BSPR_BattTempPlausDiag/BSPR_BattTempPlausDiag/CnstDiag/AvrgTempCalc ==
  BSPR_cntBattTSnsrNum : Inport
  BSPR_tBattTemp_A : Inport  Port=2
  BSPR_tBattTempMax : Inport  Port=3
  BSPR_tBattTempMin : Inport  Port=4
  Constant6 : Constant  Value=2
  Divide : Product  Inputs=*/  OutDataTypeStr=single
  Subtract : Sum  Inputs=+--  OutDataTypeStr=single
  Subtract1 : Sum  Inputs=+-  OutDataTypeStr=uint8
  SumCalc_BattTemp : Subsystem
  BSPR_tBattTempCnstAvrg : Outport
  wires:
  Constant6/1 -> Subtract1/2
  Subtract1/1 -> Divide/2
  BSPR_tBattTempMin/1 -> Subtract/3
  BSPR_tBattTempMax/1 -> Subtract/2
  Subtract/1 -> Divide/1
  Divide/1 -> BSPR_tBattTempCnstAvrg/1
  BSPR_tBattTemp_A/1 -> SumCalc_BattTemp/1(BSPR_tBattTemp_A)
  BSPR_cntBattTSnsrNum/1 -> Subtract1/1, SumCalc_BattTemp/2(BSPR_cntBattTSnsrNum)
  SumCalc_BattTemp/1(BSPR_tSumBattTemp) -> Subtract/1  "BSPR_tSumBattTemp"

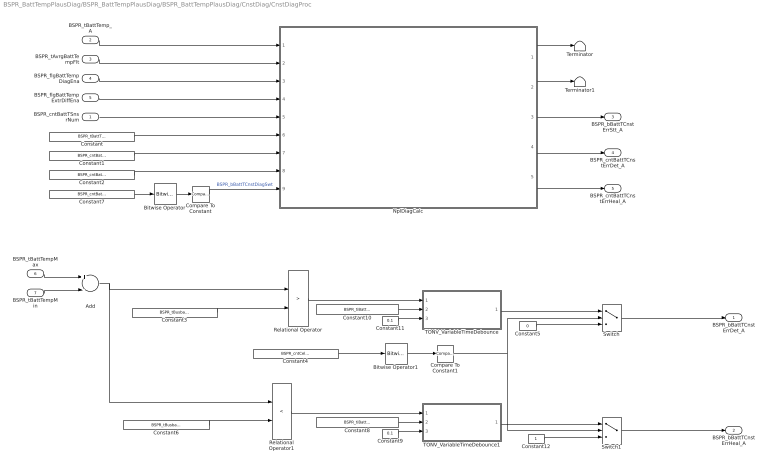
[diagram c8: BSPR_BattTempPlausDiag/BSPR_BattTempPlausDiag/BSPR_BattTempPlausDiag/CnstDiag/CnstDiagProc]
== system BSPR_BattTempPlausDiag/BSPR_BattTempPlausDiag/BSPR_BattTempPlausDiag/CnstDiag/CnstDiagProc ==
  BSPR_cntBattTSnsrNum : Inport
  BSPR_tBattTemp_A : Inport  Port=2
  BSPR_tAvrgBattTempFlt : Inport  Port=3
  BSPR_flgBattTempDiagEna : Inport  Port=4
  BSPR_flgBattTempExtrDiffEna : Inport  Port=5
  BSPR_tBattTempMax : Inport  Port=6
  BSPR_tBattTempMin : Inport  Port=7
  Add : Sum  Inputs=+-
  Bitwise Operator : simulink/Logic and Bit Operations/Bitwise Operator  logicop=AND  UseBitMask=on  BitMask=bin2dec('00000010')  BitMaskRealWorld=Stored Integer
  Bitwise Operator1 : simulink/Logic and Bit Operations/Bitwise Operator  logicop=AND  UseBitMask=on  BitMask=bin2dec('00000010')  BitMaskRealWorld=Stored Integer
  Compare To Constant : simulink/Logic and Bit Operations/Compare To Constant  relop===  const=2  OutDataTypeStr=boolean
  Compare To Constant1 : simulink/Logic and Bit Operations/Compare To Constant  relop===  const=2  OutDataTypeStr=boolean
  Constant : Constant  Value=BSPR_tBattTCnstFaultThres_C
  Constant1 : Constant  Value=BSPR_cntBattTCnstErrDet_C
  Constant10 : Constant  Value=BSPR_tiBattTCnstErrDet_C  OutDataTypeStr=single
  Constant11 : Constant  Value=0.1  OutDataTypeStr=single
  Constant12 : Constant  OutDataTypeStr=boolean
  Constant2 : Constant  Value=BSPR_cntBattTCnstErrHeal_C
  Constant3 : Constant  Value=BSPR_tBusbarTCnstFaultThres_C
  Constant4 : Constant  Value=BSPR_cntCellTPlausDiag_CW
  Constant5 : Constant  Value=0  OutDataTypeStr=boolean
  Constant6 : Constant  Value=BSPR_tBusbarTCnstHealThres_C
  Constant7 : Constant  Value=BSPR_cntBattTPlausDiag_CW
  Constant8 : Constant  Value=BSPR_tiBattTCnstErrHeal_C  OutDataTypeStr=single
  Constant9 : Constant  Value=0.1  OutDataTypeStr=single
  NplDiagCalc : Stateflow chart  TreatAsAtomicUnit=on
  Relational Operator : RelationalOperator  Operator=>  OutDataTypeStr=boolean  RndMeth=Simplest
  Relational Operator1 : RelationalOperator  Operator=<  OutDataTypeStr=boolean  RndMeth=Simplest
  Switch : Switch  Criteria=u2 > Threshold
  Switch1 : Switch  Criteria=u2 > Threshold
  TONV_VariableTimeDebounce : Subsystem  TreatAsAtomicUnit=on  RTWFcnName=TONV_VariableTimeDebounce  RTWFileName=SrvLib
  TONV_VariableTimeDebounce1 : Subsystem  TreatAsAtomicUnit=on  RTWFcnName=TONV_VariableTimeDebounce  RTWFileName=SrvLib
  Terminator : Terminator
  Terminator1 : Terminator
  BSPR_bBattTCnstErrDet_A : Outport
  BSPR_bBattTCnstErrHeal_A : Outport  Port=2
  BSPR_bBattTCnstErrStt_A : Outport  Port=3
  BSPR_cntBattTCnstErrDet_A : Outport  Port=4
  BSPR_cntBattTCnstErrHeal_A : Outport  Port=5
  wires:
  BSPR_tBattTemp_A/1 -> NplDiagCalc/1(BSPR_tBattTemp_A)
  BSPR_tAvrgBattTempFlt/1 -> NplDiagCalc/2(BSPR_tAvrgBattTempFlt)
  BSPR_flgBattTempDiagEna/1 -> NplDiagCalc/3(BSPR_flgBattTempDiagEna)
  Constant/1 -> NplDiagCalc/6(BSPR_tBattTCnstFaultThres_C)
  Constant1/1 -> NplDiagCalc/7(BSPR_cntBattTCnstErrDet_C)
  Constant2/1 -> NplDiagCalc/8(BSPR_cntBattTCnstErrHeal_C)
  BSPR_cntBattTSnsrNum/1 -> NplDiagCalc/5(BSPR_cntBattTSnsrNum)
  NplDiagCalc/3(BSPR_bBattTCnstErrStt_A) -> BSPR_bBattTCnstErrStt_A/1
  NplDiagCalc/5(BSPR_cntBattTCnstErrHeal_A) -> BSPR_cntBattTCnstErrHeal_A/1
  NplDiagCalc/4(BSPR_cntBattTCnstErrDet_A) -> BSPR_cntBattTCnstErrDet_A/1
  Compare To Constant/1 -> NplDiagCalc/9(BSPR_bBattTCnstDiagSwt)  "BSPR_bBattTCnstDiagSwt"
  Bitwise Operator/1 -> Compare To Constant/1
  Constant7/1 -> Bitwise Operator/1
  BSPR_flgBattTempExtrDiffEna/1 -> NplDiagCalc/4(BSPR_flgBattTempExtrDiffEna)
  Switch/1 -> BSPR_bBattTCnstErrDet_A/1
  TONV_VariableTimeDebounce1/1(y) -> Switch1/1
  Compare To Constant1/1 -> Switch1/2, Switch/2
  Constant4/1 -> Bitwise Operator1/1
  Relational Operator/1 -> TONV_VariableTimeDebounce/1(u)
  Constant10/1 -> TONV_VariableTimeDebounce/2(T)
  Constant11/1 -> TONV_VariableTimeDebounce/3(dT)
  Constant3/1 -> Relational Operator/2
  Add/1 -> Relational Operator1/1, Relational Operator/1
  BSPR_tBattTempMax/1 -> Add/1
  BSPR_tBattTempMin/1 -> Add/2
  Constant8/1 -> TONV_VariableTimeDebounce1/2(T)
  Constant9/1 -> TONV_VariableTimeDebounce1/3(dT)
  Switch1/1 -> BSPR_bBattTCnstErrHeal_A/1
  Constant5/1 -> Switch/3
  Constant12/1 -> Switch1/3
  TONV_VariableTimeDebounce/1(y) -> Switch/1
  Bitwise Operator1/1 -> Compare To Constant1/1
  Constant6/1 -> Relational Operator1/2
  Relational Operator1/1 -> TONV_VariableTimeDebounce1/1(u)
  NplDiagCalc/1(BSPR_bBattTCnstErrDet_A) -> Terminator/1
  NplDiagCalc/2(BSPR_bBattTCnstErrHeal_A) -> Terminator1/1

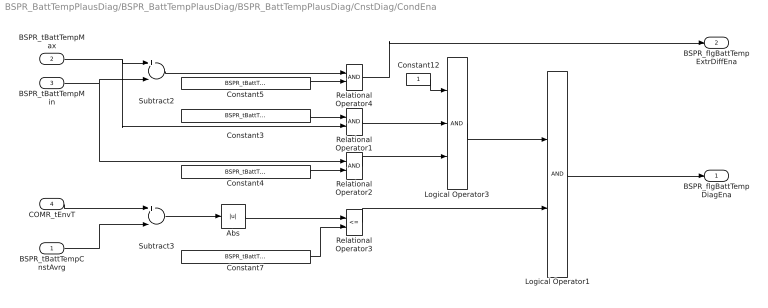
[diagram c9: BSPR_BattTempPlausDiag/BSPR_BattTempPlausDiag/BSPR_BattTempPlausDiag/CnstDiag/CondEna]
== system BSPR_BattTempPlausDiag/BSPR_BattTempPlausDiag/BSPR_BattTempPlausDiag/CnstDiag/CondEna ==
  BSPR_tBattTempCnstAvrg : Inport
  BSPR_tBattTempMax : Inport  Port=2
  BSPR_tBattTempMin : Inport  Port=3
  COMR_tEnvT : Inport  Port=4
  Abs : Abs
  Constant12 : Constant  OutDataTypeStr=boolean
  Constant3 : Constant  Value=BSPR_tBattTempCnstHi_C
  Constant4 : Constant  Value=BSPR_tBattTempCnstLo_C
  Constant5 : Constant  Value=BSPR_tBattTempCnstThres_C
  Constant7 : Constant  Value=BSPR_tBattTempEnvtDiff_C
  Logical Operator1 : Logic  AllPortsSameDT=off  OutDataTypeStr=boolean
  Logical Operator3 : Logic  Inputs=3  AllPortsSameDT=off  OutDataTypeStr=boolean
  Relational Operator1 : RelationalOperator  OutDataTypeStr=boolean  RndMeth=Simplest
  Relational Operator2 : RelationalOperator  OutDataTypeStr=boolean  RndMeth=Simplest
  Relational Operator3 : RelationalOperator  Operator=<=  OutDataTypeStr=boolean  RndMeth=Simplest
  Relational Operator4 : RelationalOperator  OutDataTypeStr=boolean  RndMeth=Simplest
  Subtract2 : Sum  Inputs=+-  OutDataTypeStr=uint8
  Subtract3 : Sum  Inputs=+-  OutDataTypeStr=single
  BSPR_flgBattTempDiagEna : Outport
  BSPR_flgBattTempExtrDiffEna : Outport  Port=2
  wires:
  BSPR_tBattTempMax/1 -> Relational Operator1/2, Subtract2/1
  BSPR_tBattTempMin/1 -> Relational Operator2/1, Subtract2/2
  Constant5/1 -> Relational Operator4/2
  Subtract2/1 -> Relational Operator4/1
  Constant3/1 -> Relational Operator1/1
  Constant4/1 -> Relational Operator2/2
  Relational Operator2/1 -> Logical Operator3/3
  COMR_tEnvT/1 -> Subtract3/1
  BSPR_tBattTempCnstAvrg/1 -> Subtract3/2
  Subtract3/1 -> Abs/1
  Constant7/1 -> Relational Operator3/2
  Logical Operator3/1 -> Logical Operator1/1
  Relational Operator3/1 -> Logical Operator1/2
  Logical Operator1/1 -> BSPR_flgBattTempDiagEna/1
  Abs/1 -> Relational Operator3/1
  Relational Operator1/1 -> Logical Operator3/2
  Relational Operator4/1 -> BSPR_flgBattTempExtrDiffEna/1
  Constant12/1 -> Logical Operator3/1

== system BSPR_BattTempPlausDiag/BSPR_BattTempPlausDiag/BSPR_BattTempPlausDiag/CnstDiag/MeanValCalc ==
  BSPR_cntBattTSnsrNum : Inport
  BSPR_tBattTemp_A : Inport  Port=2
  BSPR_tBattTempCnstAvrg : Inport  Port=3
  MeanValCalc : Stateflow chart  TreatAsAtomicUnit=on
  BSPR_tAvrgBattTempFlt : Outport
  BSPR_tSumBattTempVari : Outport  Port=2
  BSPR_tSumBattTempFlt : Outport  Port=3
  BSPR_tBattTempVari_A : Outport  Port=4
  BSPR_tAvrgBattTempVari : Outport  Port=5
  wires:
  BSPR_cntBattTSnsrNum/1 -> MeanValCalc/3(BSPR_cntBattTSnsrNum)
  MeanValCalc/3(BSPR_tSumBattTempFlt) -> BSPR_tSumBattTempFlt/1
  MeanValCalc/5(BSPR_tAvrgBattTempVari) -> BSPR_tAvrgBattTempVari/1
  MeanValCalc/2(BSPR_tSumBattTempVari) -> BSPR_tSumBattTempVari/1
  MeanValCalc/1(BSPR_tAvrgBattTempFlt) -> BSPR_tAvrgBattTempFlt/1
  MeanValCalc/4(BSPR_tBattTempVari_A) -> BSPR_tBattTempVari_A/1
  BSPR_tBattTemp_A/1 -> MeanValCalc/1(BSPR_tBattTemp_A)
  BSPR_tBattTempCnstAvrg/1 -> MeanValCalc/2(BSPR_tBattTempCnstAvrg)

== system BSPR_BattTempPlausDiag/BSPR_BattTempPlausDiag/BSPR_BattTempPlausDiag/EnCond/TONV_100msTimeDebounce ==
  note: Turn On Delay Time Deboune
  u : Inport
  T : Inport  Port=2
  Add : Sum
  Constant1 : Constant  Value=0  OutDataTypeStr=single
  Constant2 : Constant  OutDataTypeStr=uint8
  Constant3 : Constant  Value=0  OutDataTypeStr=uint8
  Constant4 : Constant  Value=0.1  OutDataTypeStr=single
  Delay : Delay  DelayLength=1  InitialCondition=0
  MinMax : MinMax  Inputs=2
  Product : Product  OutMin=[0]  OutMax=[65535]  OutDataTypeStr=single
  Relational Operator : RelationalOperator  Operator=>  OutDataTypeStr=boolean  RndMeth=Simplest
  Switch : Switch  Criteria=u2 ~= 0
  Switch1 : Switch  Criteria=u2 ~= 0
  y : Outport
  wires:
  Switch1/1 -> Product/1
  Constant3/1 -> Switch1/3
  Constant2/1 -> Switch1/1
  u/1 -> Switch1/2, Switch/2
  Constant4/1 -> Switch/1
  Constant1/1 -> Switch/3
  Add/1 -> Product/2
  Product/1 -> Relational Operator/1, Delay/1
  Switch/1 -> Add/1
  Delay/1 -> MinMax/2
  Relational Operator/1 -> y/1
  T/1 -> MinMax/1, Relational Operator/2
  MinMax/1 -> Add/2

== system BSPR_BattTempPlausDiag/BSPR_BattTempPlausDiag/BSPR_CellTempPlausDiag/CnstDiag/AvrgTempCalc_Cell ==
  BSPR_cntCellTSnsrNum : Inport
  BSPR_tCellTemp_A : Inport  Port=2
  BSPR_tCellTempMax : Inport  Port=3
  BSPR_tCellTempMin : Inport  Port=4
  Constant6 : Constant  Value=2
  Divide : Product  Inputs=*/  OutDataTypeStr=single
  Subtract : Sum  Inputs=+--  OutDataTypeStr=single
  Subtract1 : Sum  Inputs=+-  OutDataTypeStr=uint8
  SumCalc_CellTemp : Subsystem
  BSPR_tCellTempCnstAvrg : Outport
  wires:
  SumCalc_CellTemp/1(BSPR_tSumCellTemp) -> Subtract/1  "BSPR_tSumCellTemp"
  BSPR_cntCellTSnsrNum/1 -> SumCalc_CellTemp/2(BSPR_cntCellTSnsrNum), Subtract1/1
  BSPR_tCellTemp_A/1 -> SumCalc_CellTemp/1(BSPR_tCellTemp_A)
  Divide/1 -> BSPR_tCellTempCnstAvrg/1
  Subtract/1 -> Divide/1
  BSPR_tCellTempMax/1 -> Subtract/2
  BSPR_tCellTempMin/1 -> Subtract/3
  Subtract1/1 -> Divide/2
  Constant6/1 -> Subtract1/2

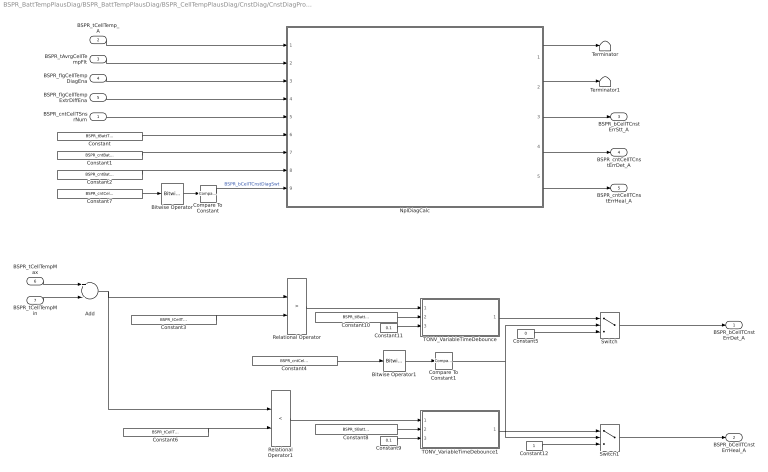
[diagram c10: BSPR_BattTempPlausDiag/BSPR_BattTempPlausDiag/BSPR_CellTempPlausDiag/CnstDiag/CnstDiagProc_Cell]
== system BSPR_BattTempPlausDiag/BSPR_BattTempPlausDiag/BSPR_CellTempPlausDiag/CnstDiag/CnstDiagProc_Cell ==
  BSPR_cntCellTSnsrNum : Inport
  BSPR_tCellTemp_A : Inport  Port=2
  BSPR_tAvrgCellTempFlt : Inport  Port=3
  BSPR_flgCellTempDiagEna : Inport  Port=4
  BSPR_flgCellTempExtrDiffEna : Inport  Port=5
  BSPR_tCellTempMax : Inport  Port=6
  BSPR_tCellTempMin : Inport  Port=7
  Add : Sum  Inputs=+-
  Bitwise Operator : simulink/Logic and Bit Operations/Bitwise Operator  logicop=AND  UseBitMask=on  BitMask=bin2dec('00000010')  BitMaskRealWorld=Stored Integer
  Bitwise Operator1 : simulink/Logic and Bit Operations/Bitwise Operator  logicop=AND  UseBitMask=on  BitMask=bin2dec('00000010')  BitMaskRealWorld=Stored Integer
  Compare To Constant : simulink/Logic and Bit Operations/Compare To Constant  relop===  const=2  OutDataTypeStr=boolean
  Compare To Constant1 : simulink/Logic and Bit Operations/Compare To Constant  relop===  const=2  OutDataTypeStr=boolean
  Constant : Constant  Value=BSPR_tBattTCnstFaultThres_C
  Constant1 : Constant  Value=BSPR_cntBattTCnstErrDet_C
  Constant10 : Constant  Value=BSPR_tiBattTCnstErrDet_C  OutDataTypeStr=single
  Constant11 : Constant  Value=0.1  OutDataTypeStr=single
  Constant12 : Constant  OutDataTypeStr=boolean
  Constant2 : Constant  Value=BSPR_cntBattTCnstErrHeal_C
  Constant3 : Constant  Value=BSPR_tCellTCnstFaultThres_C
  Constant4 : Constant  Value=BSPR_cntCellTPlausDiag_CW
  Constant5 : Constant  Value=0  OutDataTypeStr=boolean
  Constant6 : Constant  Value=BSPR_tCellTCnstHealThres_C
  Constant7 : Constant  Value=BSPR_cntCellTPlausDiag_CW
  Constant8 : Constant  Value=BSPR_tiBattTCnstErrHeal_C  OutDataTypeStr=single
  Constant9 : Constant  Value=0.1  OutDataTypeStr=single
  NplDiagCalc : Stateflow chart  TreatAsAtomicUnit=on
  Relational Operator : RelationalOperator  Operator=>  OutDataTypeStr=boolean  RndMeth=Simplest
  Relational Operator1 : RelationalOperator  Operator=<  OutDataTypeStr=boolean  RndMeth=Simplest
  Switch : Switch  Criteria=u2 > Threshold
  Switch1 : Switch  Criteria=u2 > Threshold
  TONV_VariableTimeDebounce : Subsystem  TreatAsAtomicUnit=on  RTWFcnName=TONV_VariableTimeDebounce  RTWFileName=SrvLib
  TONV_VariableTimeDebounce1 : Subsystem  TreatAsAtomicUnit=on  RTWFcnName=TONV_VariableTimeDebounce  RTWFileName=SrvLib
  Terminator : Terminator
  Terminator1 : Terminator
  BSPR_bCellTCnstErrDet_A : Outport
  BSPR_bCellTCnstErrHeal_A : Outport  Port=2
  BSPR_bCellTCnstErrStt_A : Outport  Port=3
  BSPR_cntCellTCnstErrDet_A : Outport  Port=4
  BSPR_cntCellTCnstErrHeal_A : Outport  Port=5
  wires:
  BSPR_flgCellTempExtrDiffEna/1 -> NplDiagCalc/4(BSPR_flgBattTempExtrDiffEna)
  Constant7/1 -> Bitwise Operator/1
  Bitwise Operator/1 -> Compare To Constant/1
  Compare To Constant/1 -> NplDiagCalc/9(BSPR_bBattTCnstDiagSwt)  "BSPR_bCellTCnstDiagSwt"
  NplDiagCalc/4(BSPR_cntBattTCnstErrDet_A) -> BSPR_cntCellTCnstErrDet_A/1
  NplDiagCalc/5(BSPR_cntBattTCnstErrHeal_A) -> BSPR_cntCellTCnstErrHeal_A/1
  NplDiagCalc/3(BSPR_bBattTCnstErrStt_A) -> BSPR_bCellTCnstErrStt_A/1
  BSPR_cntCellTSnsrNum/1 -> NplDiagCalc/5(BSPR_cntBattTSnsrNum)
  Constant2/1 -> NplDiagCalc/8(BSPR_cntBattTCnstErrHeal_C)
  Constant1/1 -> NplDiagCalc/7(BSPR_cntBattTCnstErrDet_C)
  Constant/1 -> NplDiagCalc/6(BSPR_tBattTCnstFaultThres_C)
  BSPR_flgCellTempDiagEna/1 -> NplDiagCalc/3(BSPR_flgBattTempDiagEna)
  BSPR_tAvrgCellTempFlt/1 -> NplDiagCalc/2(BSPR_tAvrgBattTempFlt)
  BSPR_tCellTemp_A/1 -> NplDiagCalc/1(BSPR_tBattTemp_A)
  BSPR_tCellTempMin/1 -> Add/2
  NplDiagCalc/1(BSPR_bBattTCnstErrDet_A) -> Terminator/1
  NplDiagCalc/2(BSPR_bBattTCnstErrHeal_A) -> Terminator1/1
  BSPR_tCellTempMax/1 -> Add/1
  Add/1 -> Relational Operator1/1, Relational Operator/1
  Constant3/1 -> Relational Operator/2
  Constant11/1 -> TONV_VariableTimeDebounce/3(dT)
  Constant10/1 -> TONV_VariableTimeDebounce/2(T)
  Relational Operator/1 -> TONV_VariableTimeDebounce/1(u)
  Constant4/1 -> Bitwise Operator1/1
  Bitwise Operator1/1 -> Compare To Constant1/1
  TONV_VariableTimeDebounce/1(y) -> Switch/1
  Constant5/1 -> Switch/3
  Compare To Constant1/1 -> Switch1/2, Switch/2
  Switch/1 -> BSPR_bCellTCnstErrDet_A/1
  Constant6/1 -> Relational Operator1/2
  Constant8/1 -> TONV_VariableTimeDebounce1/2(T)
  Constant9/1 -> TONV_VariableTimeDebounce1/3(dT)
  Relational Operator1/1 -> TONV_VariableTimeDebounce1/1(u)
  TONV_VariableTimeDebounce1/1(y) -> Switch1/1
  Constant12/1 -> Switch1/3
  Switch1/1 -> BSPR_bCellTCnstErrHeal_A/1
